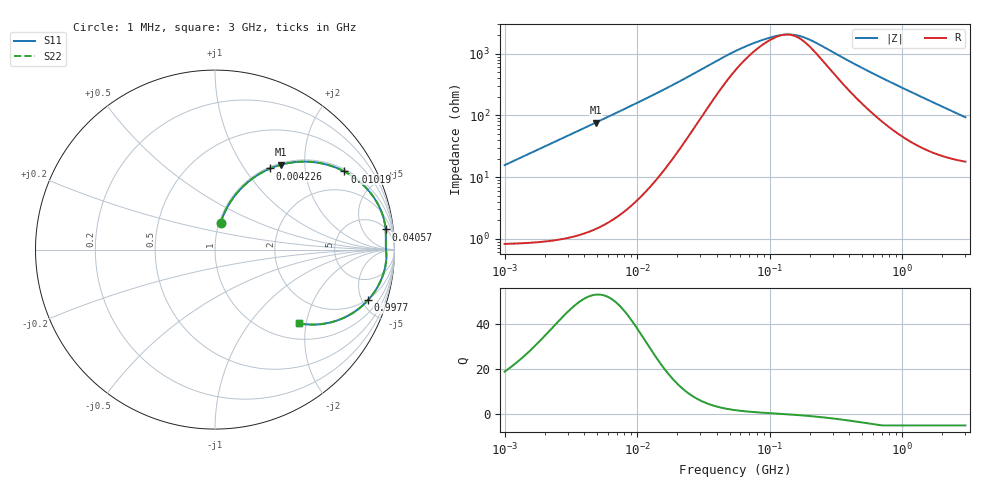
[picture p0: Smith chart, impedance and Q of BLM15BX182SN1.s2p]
! BLM15BX182SN1
# Hz S RI R 50
!Freq.(Hz) S11(Real) S11(Imag) S21(Real) S21(Imag) S12(Real) S12(Imag) S22(Real) S22(Imag)
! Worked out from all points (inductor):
!   401 points, 1 MHz to 3 GHz, reference 50 ohm
!   read as one part in series: L = 2.48 uH near 1.041 MHz
!   highest Q = 53 at 4.861 MHz (marker M1), where L = 2.49 uH
!   self-resonance near 132.3 MHz
!   S11 on the Smith chart (normalised r, x): 1 MHz: 1.02, +0.31; 4.226 MHz: 1.03, +1.32; 10.19 MHz: 1.09, +3.25; 40.57 MHz: 6, +15; 997.7 MHz: 1.91, -5.55; 3 GHz: 1.36, -1.83
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1000000  0.0313 0.1497  0.9687 -0.1497  0.9687 -0.1497  0.0313 0.1497
2139570  0.1068 0.2954  0.8932 -0.2954  0.8932 -0.2954  0.1068 0.2954
2888807  0.1746 0.3686  0.8254 -0.3686  0.8254 -0.3686  0.1746 0.3686
3823119  0.2674 0.4328  0.7326 -0.4328  0.7326 -0.4328  0.2674 0.4328
4225536  0.3077 0.452  0.6923 -0.452  0.6923 -0.452  0.3077 0.452
4861065  0.3697 0.4734  0.6303 -0.4734  0.6303 -0.4734  0.3697 0.4734
6969505  0.5461 0.4879  0.4539 -0.4879  0.4539 -0.4879  0.5461 0.4879
1.019448e7  0.7207 0.4354  0.2793 -0.4354  0.2793 -0.4354  0.7207 0.4354
1.461624e7  0.8406 0.3453  0.1594 -0.3453  0.1594 -0.3453  0.8406 0.3453
2.316168e7  0.9222 0.2235  0.0778 -0.2235  0.0778 -0.2235  0.9222 0.2235
4.05666e7  0.9507 0.1121  0.0493 -0.1121  0.0493 -0.1121  0.9507 0.1121
5.477226e7  0.952 0.0728  0.048 -0.0728  0.048 -0.0728  0.952 0.0728
8.679508e7  0.9515 0.0312  0.0485 -0.0312  0.0485 -0.0312  0.9515 0.0312
1.244416e8  0.953 0.0046  0.047 -0.0046  0.047 -0.0046  0.953 0.0046
1.614254e8  0.9544 -0.0156  0.0456 0.0156  0.0456 0.0156  0.9544 -0.0156
2.094008e8  0.9549 -0.0383  0.0451 0.0383  0.0451 0.0383  0.9549 -0.0383
4.570858e8  0.9388 -0.1329  0.0612 0.1329  0.0612 0.1329  0.9388 -0.1329
8.005644e8  0.889 -0.2354  0.111 0.2354  0.111 0.2354  0.889 -0.2354
9.977393e8  0.8517 -0.2825  0.1483 0.2825  0.1483 0.2825  0.8517 -0.2825
1.347129e9  0.778 -0.3462  0.222 0.3462  0.222 0.3462  0.778 -0.3462
1.855641e9  0.6683 -0.399  0.3317 0.399  0.3317 0.399  0.6683 -0.399
3e9  0.4706 -0.4114  0.5294 0.4114  0.5294 0.4114  0.4706 -0.4114
